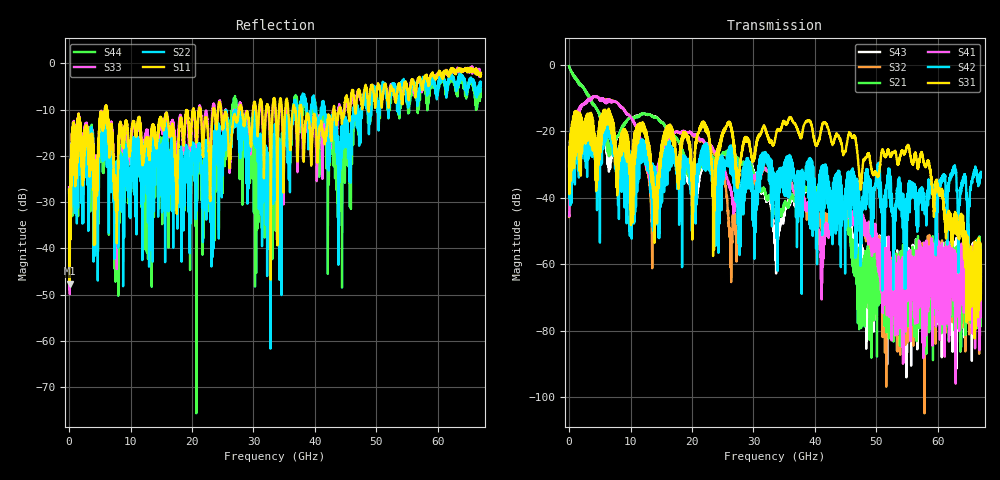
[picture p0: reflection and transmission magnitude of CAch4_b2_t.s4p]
!Agilent Technologies,N5247A,US51170199,A.09.90.13
!Agilent N5247A: A.09.90.13
!Date: Tuesday, October 23, 2018 11:22:15
!Correction: S11(Full 4 Port(1,2,3,4))
!S12(Full 4 Port(1,2,3,4))
!S13(Full 4 Port(1,2,3,4))
!S14(Full 4 Port(1,2,3,4))
!S21(Full 4 Port(1,2,3,4))
!S22(Full 4 Port(1,2,3,4))
!S23(Full 4 Port(1,2,3,4))
!S24(Full 4 Port(1,2,3,4))
!S31(Full 4 Port(1,2,3,4))
!S32(Full 4 Port(1,2,3,4))
!S33(Full 4 Port(1,2,3,4))
!S34(Full 4 Port(1,2,3,4))
!S41(Full 4 Port(1,2,3,4))
!S42(Full 4 Port(1,2,3,4))
!S43(Full 4 Port(1,2,3,4))
!S44(Full 4 Port(1,2,3,4))
!S4P File: Measurements: <S11,S12,S13,S14>,
!<S21,S22,S23,S24>,
!<S31,S32,S33,S34>,
!<S41,S42,S43,S44>:
# Hz S  dB  R 50
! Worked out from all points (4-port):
!   6701 points, 10 MHz to 67 GHz, reference 50 ohm
!   strongest paths, dB at 10 MHz, 16.76 GHz, 33.51 GHz, 50.25 GHz, 67 GHz:
!     S31: -30.6, -22.7, -22.5, -33.5, -68.8
!     S42: -30.8, -26.9, -33.6, -36.7, -32.2
!     S41: -45.5, -20.9, -33.8, -54.7, -65.2
!     S21: -0.4, -21.1, -44.4, -58.4, -63.5
!     S32: -45.8, -21.0, -33.6, -53.3, -62.4
!     S43: -0.4, -21.2, -52.0, -55.3, -60.9
!   lowest |S11| = -47.6 dB at 79.99 MHz (marker M1), VSWR 1.01, Z = 49.7 - j0.322 ohm
!   |S11| at or under -10 dB: start of sweep to 5.852 GHz; 6.189 GHz to 20.16 GHz (13.97 GHz wide, 106 % of centre); 37.86 GHz to 43.04 GHz (5.181 GHz wide, 12.8 % of centre)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
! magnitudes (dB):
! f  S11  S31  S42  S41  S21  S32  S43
! 10 MHz  -27.2  -30.6  -30.8  -45.5  -0.4  -45.8  -0.4
! 79.99 MHz  -47.6  -25.2  -25.7  -39.1  -0.9  -39.3  -0.9
! 7.459 GHz  -26.3  -23.7  -27.7  -11.1  -23.1  -11.1  -23.5
! 13.55 GHz  -13.2  -32.6  -48.8  -38.4  -15.6  -56.6  -15.5
! 19.57 GHz  -15.9  -23.0  -28.5  -20.2  -33.6  -20.3  -35.9
! 55.09 GHz  -6.0  -24.3  -43.8  -57.0  -61.3  -66.4  -61.3
! 67 GHz  -2.1  -68.8  -32.2  -65.2  -63.5  -62.4  -60.9
